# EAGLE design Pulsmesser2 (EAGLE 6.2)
Pulsmesser
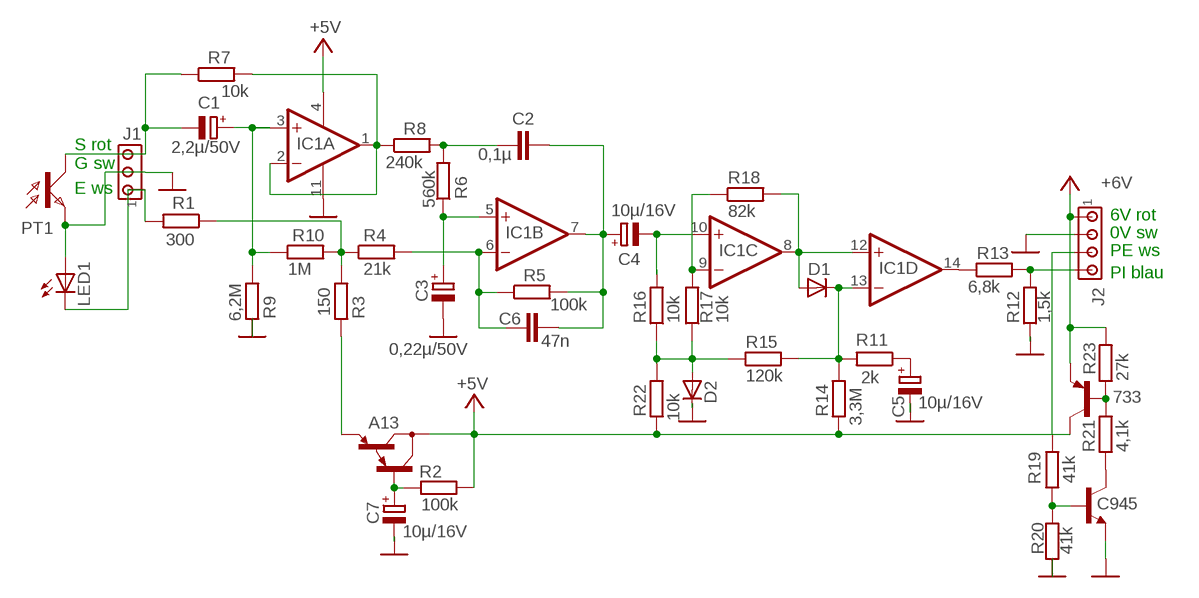
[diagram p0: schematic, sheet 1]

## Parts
733  -PNP-TO92-ECB  [TO92-ECB]
A13  MPSA65  [TO92-CBE]
C1  2,2µ/50V  CPOL-EUE1.8-4  [E1,8-4]
C2  0,1µ  C-EU050-024X044  [C050-024X044]
C3  0,22µ/50V  CPOL-EUE1.8-4  [E1,8-4]
C4  10µ/16V  CPOL-EUE1.8-4  [E1,8-4]
C5  10µ/16V  CPOL-EUE1.8-4  [E1,8-4]
C6  47n  C-EU025-024X044  [C025-024X044]
C7  10µ/16V  CPOL-EUE1.8-4  [E1,8-4]
C945  2SC945  [TO92-ECB@1]
D1  1N4148DO35-7  [DO35-7]
D2  1N4148DO35-7  [DO35-7]
IC1  LM324N  [DIL14]
J1  MTA03-100  [10X03MTA]
J2  MTA04-100  [10X04MTA]
LED1  LED3MM  [LED3MM]
PT1  BPX81  [BPX81]
R1  300  R-EU_0204/7  [0204/7]
R2  100k  R-EU_0204/7  [0204/7]
R3  150  R-EU_0204/7  [0204/7]
R4  21k  R-EU_0204/7  [0204/7]
R5  100k  R-EU_0204/7  [0204/7]
R6  560k  R-EU_0204/7  [0204/7]
R7  10k  R-EU_0204/7  [0204/7]
R8  240k  R-EU_0204/7  [0204/7]
R9  6,2M  R-EU_0204/7  [0204/7]
R10  1M  R-EU_0204/7  [0204/7]
R11  2k  R-EU_0204/7  [0204/7]
R12  1,5k  R-EU_0204/7  [0204/7]
R13  6,8k  R-EU_0204/7  [0204/7]
R14  3,3M  R-EU_0204/7  [0204/7]
R15  120k  R-EU_0204/7  [0204/7]
R16  10k  R-EU_0204/7  [0204/7]
R17  10k  R-EU_0204/7  [0204/7]
R18  82k  R-EU_0204/7  [0204/7]
R19  41k  R-EU_0204/7  [0204/7]
R20  41k  R-EU_0204/7  [0204/7]
R21  4,1k  R-EU_0204/7  [0204/7]
R22  10k  R-EU_0204/7  [0204/7]
R23  27k  R-EU_0204/7  [0204/7]

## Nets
+5V: 733.C A13.C IC1.4(P:V+) R2.2 R14.1 R22.1
+6V: 733.E J2.1 R23.2
GND: C3.- C5.- C7.- C945.E D2.C IC1.11(P:V-) J1.2 J2.2 LED1.A PT1.E R9.2 R12.1 R20.1
N$1: C2.1 R6.2 R8.2
N$2: C1.+ IC1.3(A:+IN) R9.1 R10.1
N$3: C2.2 C4.+ C6.2 IC1.7(B:OUT) R5.2
N$4: C4.- IC1.10(C:+IN) R16.2
N$5: IC1.9(C:-IN) R17.2 R18.1
N$6: D1.A IC1.8(C:OUT) IC1.12(D:+IN) R18.2
N$7: C3.+ IC1.5(B:+IN) R6.1
N$8: A13.E R3.2
N$9: C6.1 IC1.6(B:-IN) R4.2 R5.1
N$10: IC1.1(A:OUT) IC1.2(A:-IN) R7.2 R8.1
N$11: D1.C IC1.13(D:-IN) R11.2 R14.2 R15.2
N$12: J2.4 R12.2 R13.2
N$13: IC1.14(D:OUT) R13.1
N$14: C5.+ R11.1
N$15: D2.A R15.1 R16.1 R17.1 R22.2
N$16: J1.1 LED1.K(C) R1.2
N$18: R1.1 R3.1 R4.1 R10.2
N$19: A13.B C7.+ R2.1
N$20: 733.B R21.2 R23.1
N$21: C945.C R21.1
N$23: J2.3 R19.2
N$24: C945.B R19.1 R20.2
R7: C1.- J1.3 PT1.C R7.1

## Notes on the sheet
- S rot
- G sw
- E ws
- 6V rot
- 0V sw
- PE ws
- PI blau

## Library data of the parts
733 = transistor-neu-to92:*-PNP-: PNP Transistror
A13 = transistor-pnp:MPSA65*: PNP Darlington Transistor Source: http://www.fairchildsemi.com/ds/MP/MPSA65.pdf
C1 C3-C5 C7 = rcl:CPOL-EU: POLARIZED CAPACITOR, European symbol
C2 C6 = rcl:C-EU: CAPACITOR, European symbol
C945 = transistor:2SC945: NPN Silicon Epitaxial Planar Transistor Source: SEMTECH ELECTRONICS LTD. ... 2SC945 2.pdf
D1 D2 = diode:1N4148: DIODE
IC1 = linear:LM324: OP AMP
J1 = con-amp:MTA03-100: AMP connector
J2 = con-amp:MTA04-100: AMP connector
LED1 = led:LED: LED
PT1 = opto-trans-siemens:BPX81: PHOTO TRANSISTOR; OC_FARNELL: unknown; OC_NEWARK: unknown
R1-R23 = rcl:R-EU_: RESISTOR, European symbol

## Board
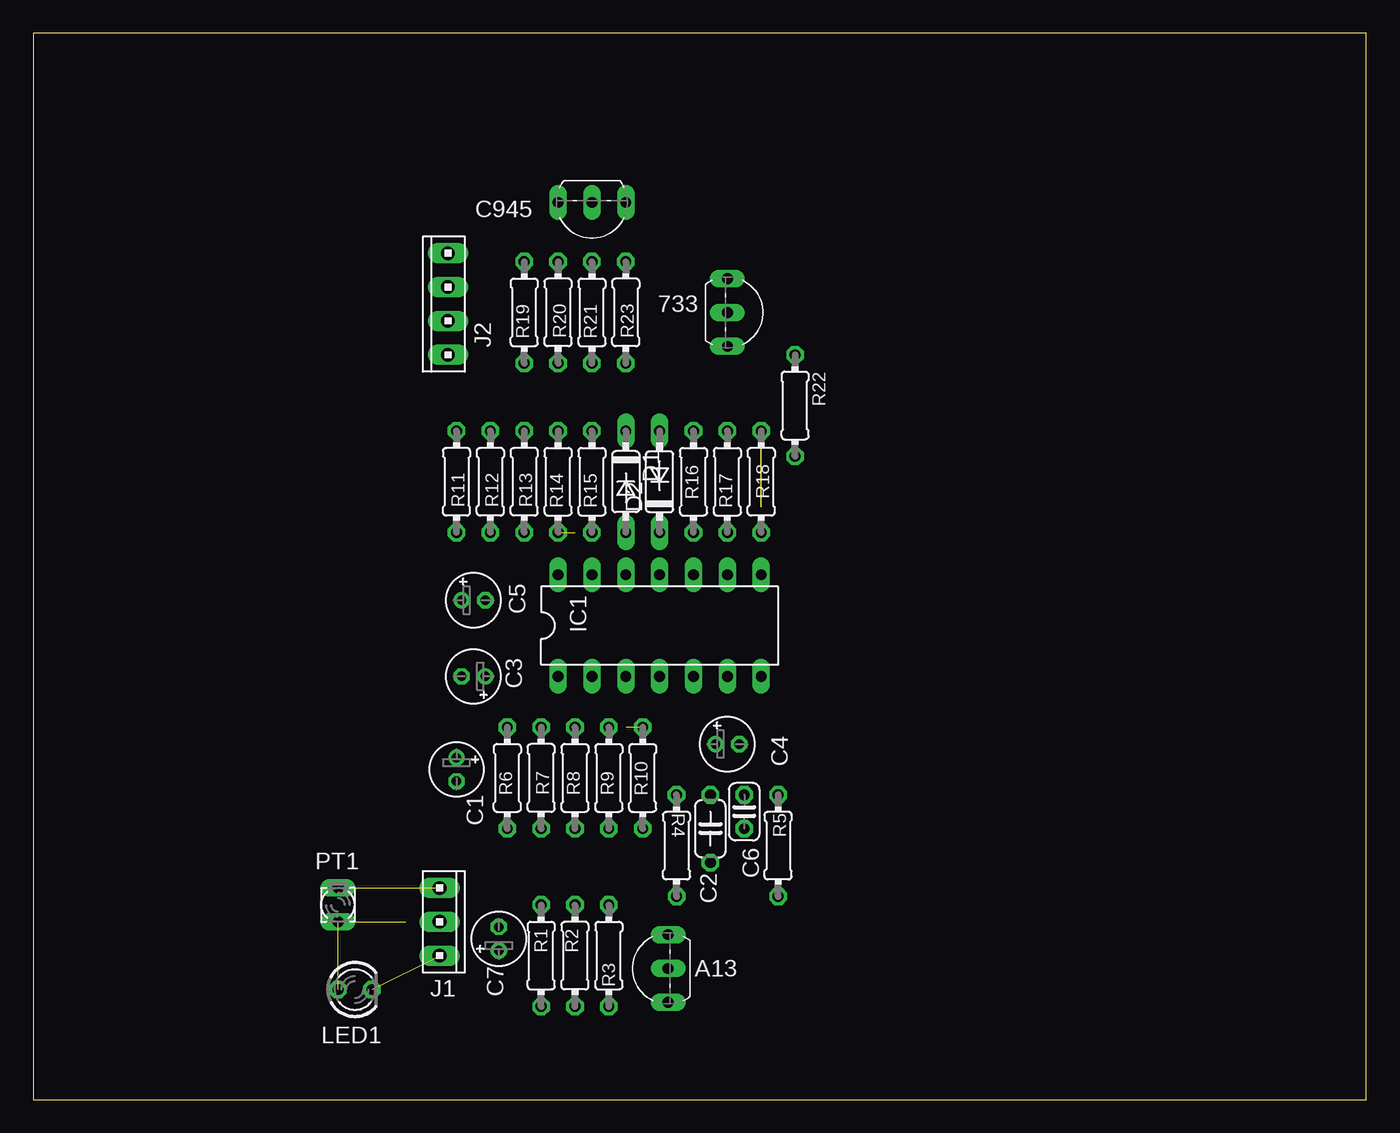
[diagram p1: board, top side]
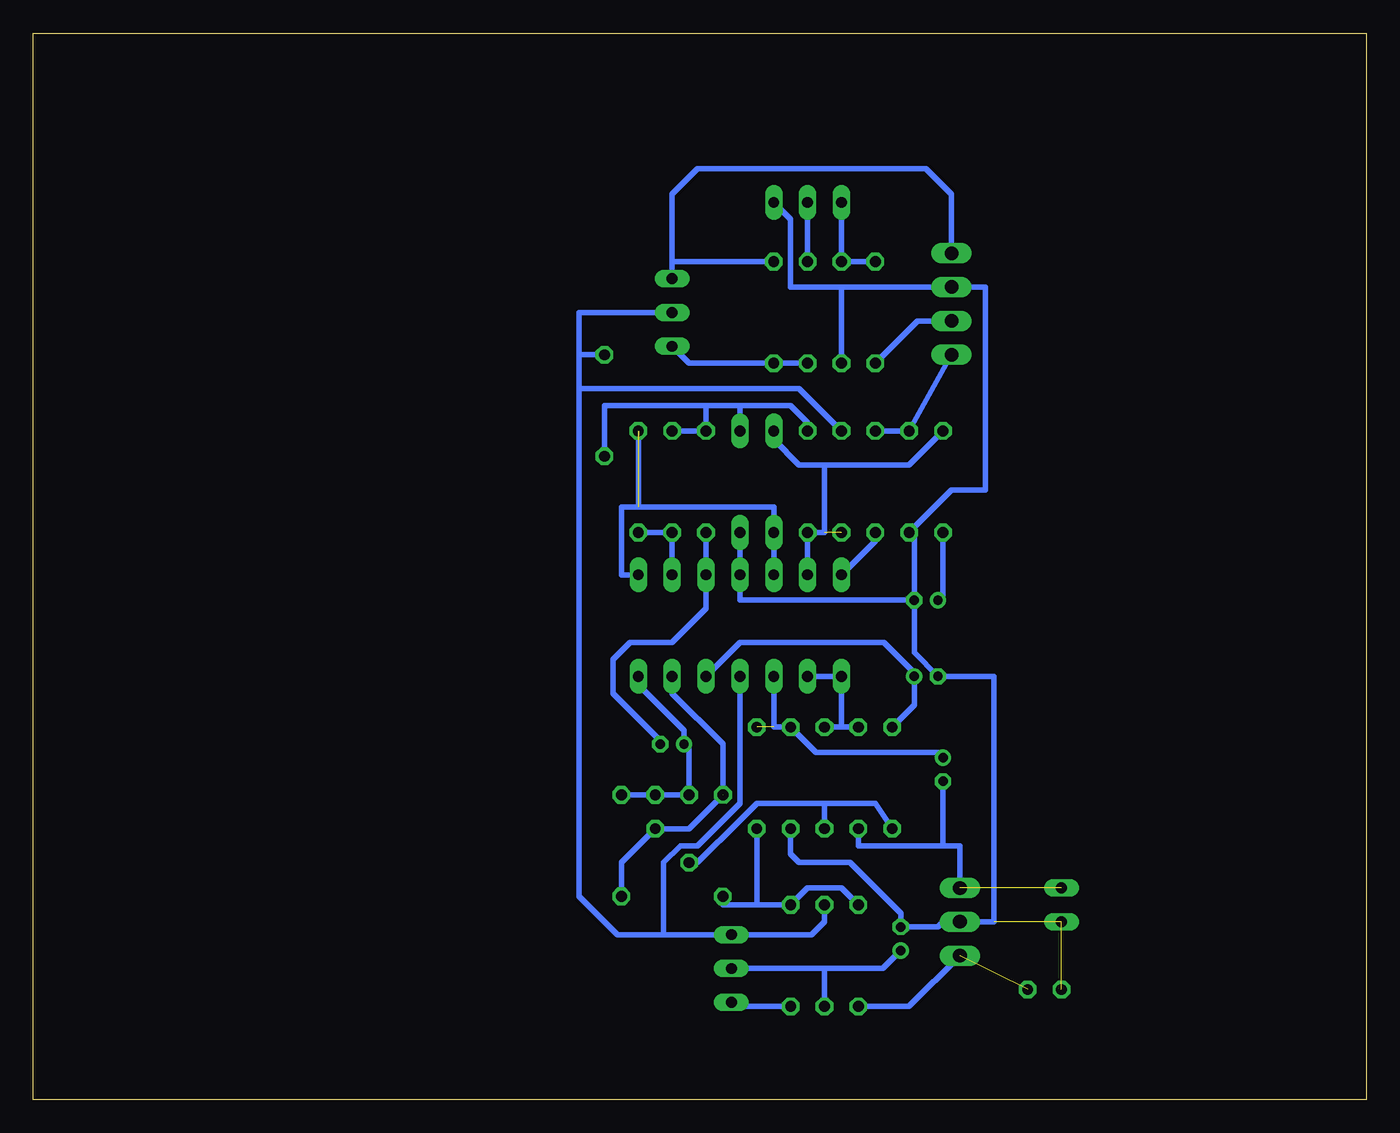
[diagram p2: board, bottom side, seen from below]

Size 100 x 80 mm. Coordinates in mm from the lower left corner, seen from the top.
Outline: 0,0 100,0 100,80 0,80 0,0
Copper layers (1*16): Top 0.035mm / dielectric 1.5mm / Bottom 0.035mm
Design rules: minimum track width 10mil, minimum drill 24mil, track to track 8mil, track to pad 8mil, pad to pad 8mil, via to via 8mil, smd to smd 8mil, copper to edge 40mil, drill to drill 8mil, minimum pad ring 10mil, minimum via ring 8mil, stop-mask expansion 4mil, vias tented up to drill 0mil, thermal gap 10mil

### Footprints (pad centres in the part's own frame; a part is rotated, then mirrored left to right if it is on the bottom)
TO92-ECB = drill 0.813 long: B 2.54,0; C 0,0; E -2.54,0
TO92-CBE = drill 0.813 long: B 0,0; C 2.54,0; E -2.54,0
E1,8-4 = drill 0.711 pad 1.168: + -0.889,0 | drill 0.711 pad 1.168 octagon: - 0.889,0
C050-024X044 = drill 0.813 octagon: 1 -2.54,0; 2 2.54,0
C025-024X044 = drill 0.813 octagon: 1 -1.27,0; 2 1.27,0
DO35-7 = drill 0.813 long: A 3.81,0; C -3.81,0
DIL14 = drill 0.813 long: 1 -7.62,-3.81; 2 -5.08,-3.81; 3 -2.54,-3.81; 4 0,-3.81; 5 2.54,-3.81; 6 5.08,-3.81; 7 7.62,-3.81; 8 7.62,3.81; 9 5.08,3.81; 10 2.54,3.81; 11 0,3.81; 12 -2.54,3.81; 13 -5.08,3.81; 14 -7.62,3.81
10X03MTA = drill 1.016 long: 1 2.54,0; 2 0,0; 3 -2.54,0
10X04MTA = drill 1.016 long: 1 3.81,0; 2 1.27,0; 3 -1.27,0; 4 -3.81,0
LED3MM = drill 0.813 octagon: A -1.27,0; K 1.27,0
BPX81 = drill 0.813 long: C 1.27,0; E -1.27,0
0204/7 = drill 0.813 octagon: 1 -3.81,0; 2 3.81,0

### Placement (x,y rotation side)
733  52.07,59.05 270 top
A13  47.62,9.83 90 top
C1  31.75,24.77 270 top
C2  50.8,20.32 90 top
C3  33.02,31.75 180 top
C4  52.07,26.67 0 top
C5  33.02,37.47 0 top
C6  53.34,21.59 90 top
C7  34.92,12.06 90 top
C945  [TO92-ECB]  41.91,67.31 180 top
D1  44.45,46.35 270 top
D2  46.99,46.35 90 top
IC1  46.99,35.56 0 top
J1  30.48,13.34 270 top
J2  31.11,59.69 90 top
LED1  24.13,8.26 0 top
PT1  22.86,14.61 90 top
R1  38.1,10.79 270 top
R2  40.64,10.79 90 top
R3  43.18,10.79 270 top
R4  48.26,19.05 90.1 top
R5  55.88,19.05 90 top
R6  35.56,24.13 270 top
R7  38.1,24.13 90 top
R8  40.64,24.13 270 top
R9  43.18,24.13 270 top
R10  45.72,24.13 270 top
R11  31.75,46.35 90 top
R12  34.29,46.35 90 top
R13  36.83,46.35 90 top
R14  39.37,46.35 270 top
R15  41.91,46.35 270 top
R16  49.53,46.35 270 top
R17  52.07,46.35 270 top
R18  54.61,46.35 90 top
R19  36.83,59.05 270 top
R20  39.37,59.05 90 top
R21  41.91,59.05 270 top
R22  57.15,52.07 270 top
R23  44.45,59.05 90 top

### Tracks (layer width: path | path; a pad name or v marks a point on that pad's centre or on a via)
+5V
  Bottom 0.406: R2.2 40.64,13.34 41.6,12.37 A13.C 52.7,12.37 | IC1.4 46.99,22.23 50.16,19.05 51.44,19.05 52.7,17.78 52.7,12.37 | R14.1 42.55,53.34 57.15,53.34 59.05,53.34 | 59.05,55.88 59.05,53.34 | 59.05,53.34 59.05,15.24 56.19,12.37 52.7,12.37 | R22.1 59.05,55.88 | 59.05,55.88 59.05,59.05 733.C
+6V
  Bottom 0.406: J2.1 31.11,67.94 33.02,69.85 50.16,69.85 52.07,67.94 52.07,62.87 | 52.07,62.87 733.E | R23.2 52.07,62.87
GND  (2 unrouted)
  Bottom 0.406: R9.2 43.18,18.41 42.55,17.78 38.73,17.78 34.92,13.97 C7.- 32.13,12.95 31.75,13.34 J1.2 27.94,13.34 27.94,31.75 C3.- 33.91,33.53 C5.- | C945.E 43.18,66.04 43.18,60.96 39.37,60.96 | 39.37,60.96 J2.2 28.57,60.96 28.57,45.72 31.11,45.72 R12.1 33.91,42.16 C5.- | IC1.11 D2.C 46.99,37.47 C5.- | 39.37,60.96 R20.1
N$1
  Bottom 0.406: R6.2 36.83,22.23 40.64,22.23 | 40.64,22.23 R8.2 | C2.1 50.16,17.78 46.99,20.95 | 46.99,20.95 45.72,22.23 | 45.72,22.23 46.99,20.95 | 46.99,20.95 45.72,22.23 | 45.72,22.23 40.64,22.23
N$2  (1 unrouted)
  Bottom 0.406: IC1.3 44.45,27.94 R9.1 41.27,26.04 32.13,26.04 C1.+
N$3
  Bottom 0.406: R5.2 C6.2 C2.2 50.8,26.29 C4.+ 51.18,27.69 54.61,31.11 IC1.7
N$4
  Bottom 0.406: 49.53,36.83 IC1.10 R16.2 | 49.53,36.83 49.53,37.47 49.53,36.83 | 49.53,36.83 50.8,35.56 52.07,34.29 55.24,34.29 56.52,33.02 56.52,30.48 52.96,26.92 C4.-
N$5
  Bottom 0.406: R18.1 R17.2 IC1.9
N$6  (2 unrouted)
  Bottom 0.406: IC1.8 55.88,39.37 55.88,44.45 54.61,44.45 | 54.61,44.45 R18.2 | D1.A IC1.12 44.45,44.45 54.61,44.45
N$7
  Bottom 0.406: R6.1 33.91,29.59 C3.+ 33.91,32 36.2,34.29 46.99,34.29 IC1.5
N$8
  Bottom 0.406: R3.2 47.32,6.99 A13.E
N$9  (1 unrouted)
  Bottom 0.406: IC1.6 52.07,30.48 48.26,26.67 R4.2 50.8,20.32 C6.1 55.88,17.78 R5.1
N$10
  Bottom 0.406: R7.2 39.37,27.94 | 39.37,27.94 R8.1 39.37,27.94 | IC1.1 IC1.2 IC1.1 | 39.37,27.94 IC1.1
N$11  (1 unrouted)
  Bottom 0.406: R11.2 34.29,47.62 40.64,47.62 | 40.64,47.62 42.55,47.62 44.45,49.53 D1.C | 40.64,42.55 R15.2 | R15.2 IC1.13 | R15.2 40.64,42.55 | 40.64,42.55 40.64,47.62
N$12
  Bottom 0.406: R13.2 R12.2 J2.4
N$13
  Bottom 0.406: IC1.14 36.83,41.91 R13.1
N$14
  Bottom 0.406: R11.1 31.75,37.85 C5.+
N$15
  Bottom 0.406: R17.1 R16.1 49.53,52.07 | 47.62,52.07 46.99,52.07 | 46.99,52.07 43.18,52.07 41.91,50.8 R15.1 | 47.62,52.07 46.99,52.07 | 46.99,52.07 D2.A | D2.A 46.99,49.53 D2.A | 49.53,52.07 47.62,52.07 | R22.2 57.15,52.07 54.61,52.07 49.53,52.07
N$16  (1 unrouted)
  Bottom 0.406: R1.2 34.29,6.99 J1.1
N$18
  Bottom 0.406: 45.72,14.61 R3.1 41.91,15.88 40.64,15.88 39.37,15.88 R1.1 | 45.72,14.61 R10.2 | 45.72,14.61 48.27,14.61 R4.1
N$19
  Bottom 0.406: A13.B 40.95,9.83 | C7.+ 36.27,9.83 40.95,9.83 | 40.95,9.83 40.64,9.83 R2.1
N$20
  Bottom 0.406: R21.2 R23.1 50.8,55.24 733.B
N$21
  Bottom 0.406: R21.1 C945.C
N$23
  Bottom 0.406: J2.3 33.66,58.42 R19.2
N$24
  Bottom 0.406: R19.1 R20.2 C945.B
R7  (1 unrouted)
  Bottom 0.406: 30.48,19.05 31.75,19.05 | 31.75,19.05 38.1,19.05 R7.1 | J1.3 30.48,19.05 | 30.48,19.05 31.75,19.05 | 31.75,19.05 C1.-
